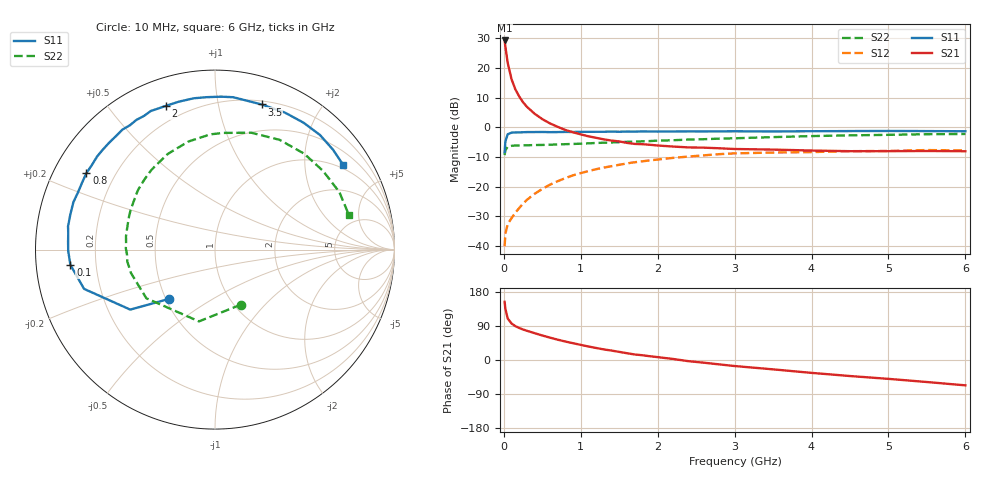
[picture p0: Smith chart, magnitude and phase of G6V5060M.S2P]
! SIEMENS Small Signal Semiconductors
! BFG193
! Si NPN RF Bipolar Junction Transistor in SOT223
! VCE = 0.5 V  IC = 60 mA
! Common Emitter S-Parameters:  August  1996
# GHz  S  MA  R  50
!  f  S11  S21  S12  S22
! GHz  MAG  ANG  MAG  ANG  MAG  ANG  MAG  ANG
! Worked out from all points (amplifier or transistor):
!   36 points, 10 MHz to 6 GHz, reference 50 ohm
!   highest |S21| = 29.3 dB at 10 MHz (marker M1)
!   |S21| within 3 dB of that: start of sweep to 25.17 MHz
!   unconditionally stable (mu >= 1): start of sweep to 17.19 MHz; 104.5 MHz to end of sweep
!   at 250 MHz: K = 1.30, MAG = 13.8 dB, |S12| = -25.7 dB
!   at 1.4 GHz: K = 1.26, MAG = 1.2 dB, |S12| = -13.1 dB
!   at 6 GHz: K = 1.08, MAG = -1.8 dB, |S12| = -7.8 dB
!   S11 on the Smith chart (normalised r, x): 10 MHz: 0.52, -0.33; 100 MHz: 0.11, -0.05; 800 MHz: 0.10, +0.27; 2 GHz: 0.12, +0.71; 3.5 GHz: 0.23, +1.35; 6 GHz: 0.87, +3.10
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0.01  0.3778 -133.2  29.02 153.4  0.0099 61.0  0.3388 -64.9
0.02  0.5786 -144.7  22.91 135.0  0.016 51.0  0.4098 -102.6
0.05  0.7617 -163.3  12.17 109.6  0.0233 40.9  0.4689 -144.7
0.1  0.8103 -174.0  6.454 96.4  0.0294 45.5  0.4859 -164.4
0.15  0.8179 -179.5  4.342 89.3  0.0363 51.3  0.4933 -172.3
0.2  0.8198 176.9  3.296 84.5  0.0436 55.3  0.491 -176.9
0.25  0.8226 173.7  2.633 80.5  0.0516 57.8  0.497 179.2
0.3  0.829 171.0  2.21 77.1  0.0598 59.2  0.4962 176.5
0.4  0.8295 166.3  1.689 70.8  0.0755 60.2  0.5015 171.4
0.5  0.832 161.5  1.37 64.7  0.0912 59.3  0.5033 166.9
0.6  0.8274 157.5  1.16 59.0  0.1078 58.5  0.5072 163.1
0.8  0.8337 149.3  0.9 48.7  0.139 54.0  0.5182 155.6
1.1  0.8372 138.4  0.703 35.7  0.1825 47.2  0.5356 145.3
1.3  0.8393 131.0  0.625 27.9  0.2091 41.9  0.5484 138.1
1.6  0.8449 121.2  0.545 17.9  0.2456 33.4  0.5677 128.7
2  0.8465 109.0  0.492 7.6  0.2858 22.5  0.5944 116.2
2.2  0.8484 103.7  0.473 2.7  0.3045 17.1  0.6038 110.0
2.8  0.8527 87.7  0.442 -11.6  0.3518 1.4  0.6426 92.2
3.5  0.8493 72.2  0.42 -24.7  0.3744 -17.0  0.6819 72.7
4.5  0.8621 55.1  0.395 -42.3  0.3954 -35.5  0.7295 47.1
5.5  0.8614 40.3  0.398 -58.1  0.4125 -56.2  0.7633 24.9
6  0.8563 33.5  0.394 -66.9  0.4059 -67.8  0.7704 14.6
